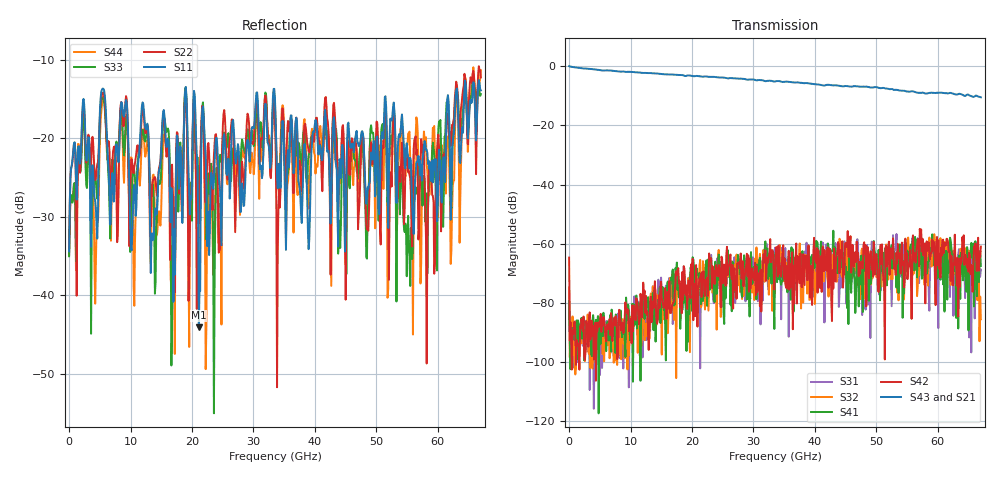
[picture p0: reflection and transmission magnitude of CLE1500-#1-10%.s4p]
!Keysight Technologies,N5247B,US50470101,A.16.20.02
!Date: Thursday, March 13, 2025 10:10:35
!Correction: S11(C  4-Port  )
!S12(C  4-Port  )
!S13(C  4-Port  )
!S14(C  4-Port  )
!S21(C  4-Port  )
!S22(C  4-Port  )
!S23(C  4-Port  )
!S24(C  4-Port  )
!S31(C  4-Port  )
!S32(C  4-Port  )
!S33(C  4-Port  )
!S34(C  4-Port  )
!S41(C  4-Port  )
!S42(C  4-Port  )
!S43(C  4-Port  )
!S44(C  4-Port  )
!S4P File: Measurements: <S11,S12,S13,S14>,
!<S21,S22,S23,S24>,
!<S31,S32,S33,S34>,
!<S41,S42,S43,S44>:
# Hz S  dB  R 50
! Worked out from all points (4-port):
!   601 points, 10 MHz to 67 GHz, reference 50 ohm
!   strongest paths, dB at 10 MHz, 16.76 GHz, 33.51 GHz, 50.25 GHz, 67 GHz:
!     S43: 0.0, -2.8, -5.2, -7.2, -10.5
!     S21: 0.0, -2.9, -5.3, -7.3, -10.7
!     S42: -64.7, -80.8, -69.1, -75.8, -61.0
!     S41: -79.4, -72.2, -71.3, -68.0, -67.5
!     S32: -74.9, -70.7, -69.0, -68.8, -85.5
!     S31: -76.2, -69.3, -61.3, -70.3, -68.8
!   lowest |S11| = -44.1 dB at 21.11 GHz (marker M1), VSWR 1.01, Z = 49.8 + j0.575 ohm
!   |S11| at or under -10 dB: start of sweep to end of sweep
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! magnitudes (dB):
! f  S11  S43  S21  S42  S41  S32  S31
! 10 MHz  -34.4  0.0  0.0  -64.7  -79.4  -74.9  -76.2
! 5.481 GHz  -13.6  -1.5  -1.6  -87.8  -91.3  -97.4  -95.4
! 16.87 GHz  -33.8  -2.8  -2.9  -80.3  -68.7  -75.2  -87.2
! 21.11 GHz  -44.1  -3.3  -3.5  -74.0  -71.7  -74.8  -75.4
! 51.15 GHz  -20.0  -7.3  -7.5  -72.4  -63.1  -67.6  -67.0
! 55.61 GHz  -22.9  -8.5  -8.3  -71.6  -60.3  -62.7  -63.5
! 67 GHz  -13.9  -10.5  -10.7  -61.0  -67.5  -85.5  -68.8
